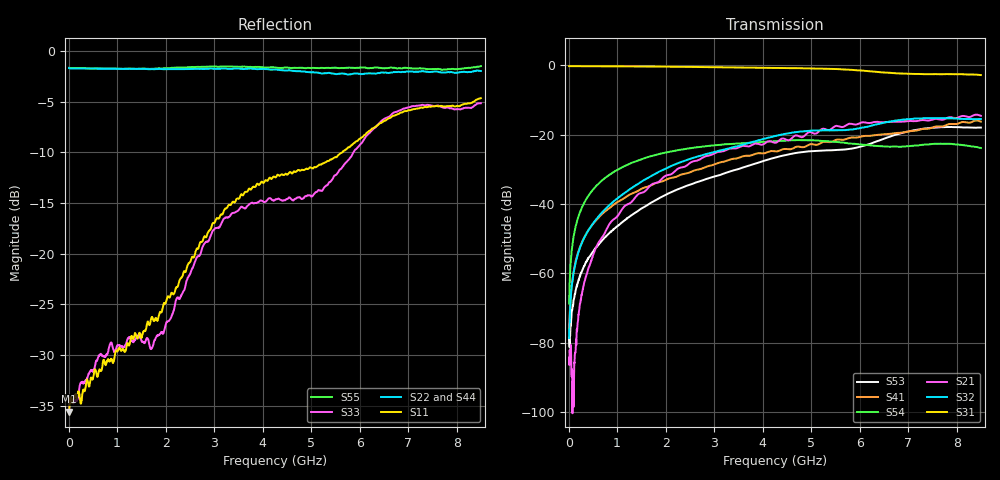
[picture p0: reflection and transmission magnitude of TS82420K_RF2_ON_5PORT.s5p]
!Created with skrf (http://scikit-rf.org).
# GHz S RI R 50.0
!freq ReS11 ImS11 ReS12 ImS12 ReS13 ImS13
! ReS14 ImS14 ReS15 ImS15
! ReS21 ImS21 ReS22 ImS22 ReS23 ImS23
! ReS24 ImS24 ReS25 ImS25
! ReS31 ImS31 ReS32 ImS32 ReS33 ImS33
! ReS34 ImS34 ReS35 ImS35
! ReS41 ImS41 ReS42 ImS42 ReS43 ImS43
! ReS44 ImS44 ReS45 ImS45
! ReS51 ImS51 ReS52 ImS52 ReS53 ImS53
! ReS54 ImS54 ReS55 ImS55
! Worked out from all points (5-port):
!   1601 points, 10 MHz to 8.5 GHz, reference 50 ohm
!   strongest paths, dB at 10 MHz, 2.132 GHz, 4.255 GHz, 6.378 GHz, 8.5 GHz:
!     S31: -0.2, -0.4, -0.7, -1.9, -2.8
!     S32: -78.7, -28.9, -20.4, -16.9, -15.5
!     S21: -84.4, -31.3, -22.3, -16.3, -14.5
!     S54: -68.8, -24.8, -21.9, -23.3, -23.8
!     S41: -75.9, -32.4, -24.8, -20.0, -16.2
!     S53: -78.6, -36.5, -26.6, -21.8, -17.9
!   lowest |S11| = -35.6 dB at 10 MHz (marker M1), VSWR 1.03, Z = 51.7 + j0.0169 ohm
!   |S11| at or under -10 dB: start of sweep to 5.639 GHz
